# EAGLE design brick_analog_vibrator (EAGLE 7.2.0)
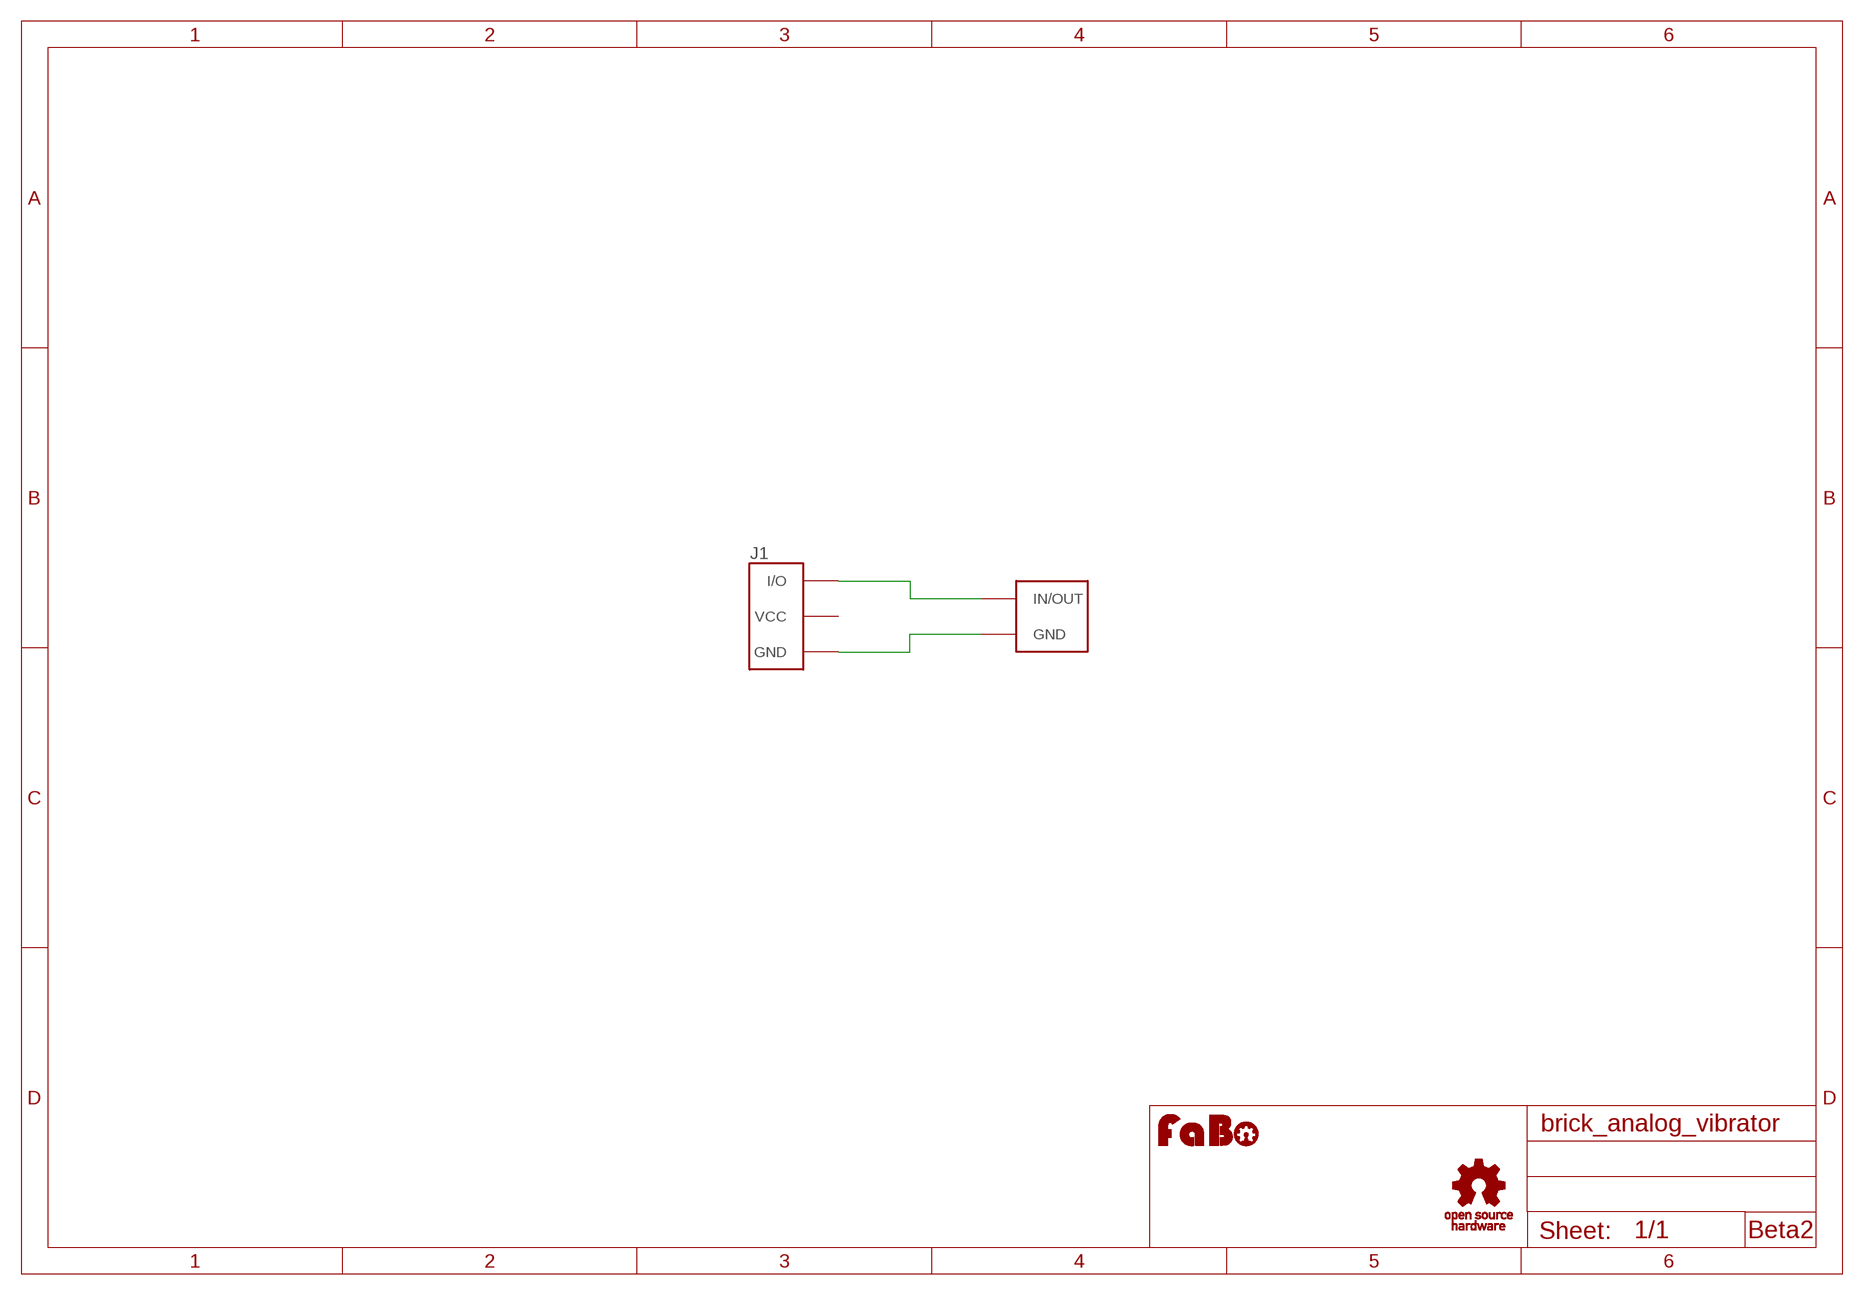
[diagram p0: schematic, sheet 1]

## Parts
J1  BRICK_3PIN  [BRICK_3PIN]
U1  LA3R5-480H1-PTH  [LA3R5-480AH1_PTH]
U$1  LOGO_FABO-M  [LOGO_FABO_M]
U$5  LOGO_OSHW_T-M  [LOGO_OSHW_T_M]

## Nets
GND: J1.GND U1.P$2(GND)
N$1: J1.IN/OUT(I/O) U1.P$1(IN/OUT)
Unconnected: J1.VCC

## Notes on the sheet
- Beta2

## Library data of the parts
J1 = gclue:BRICK_3PIN: FaBo Brick 3pin
U1 = gclue:LA3R5-480H1
U$1 = FaBo:LOGO_FABO
U$5 = gclue:LOGO_OSHW_T

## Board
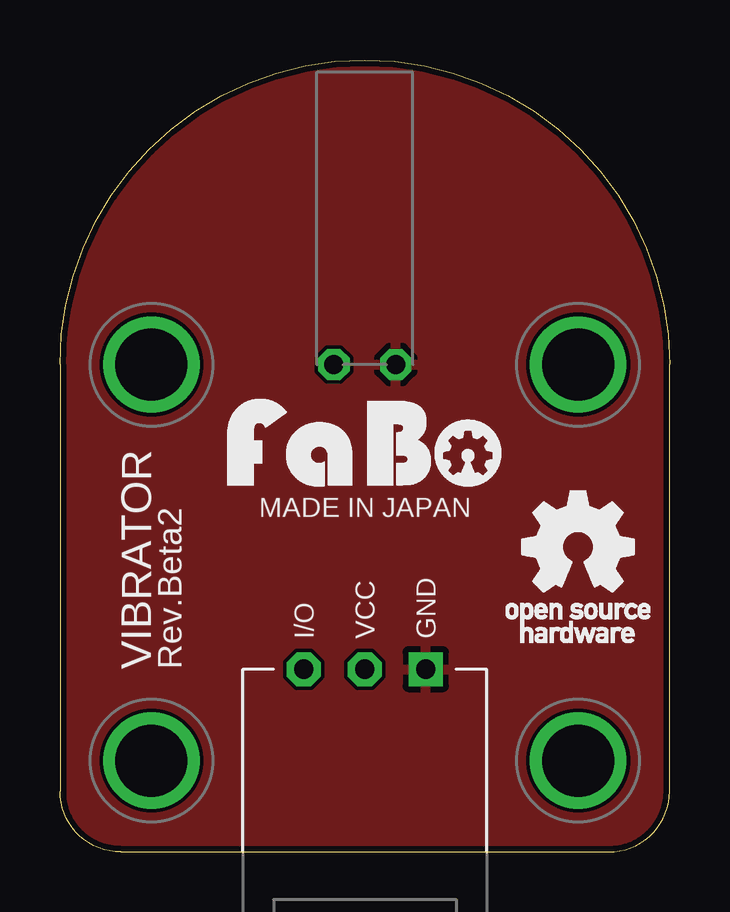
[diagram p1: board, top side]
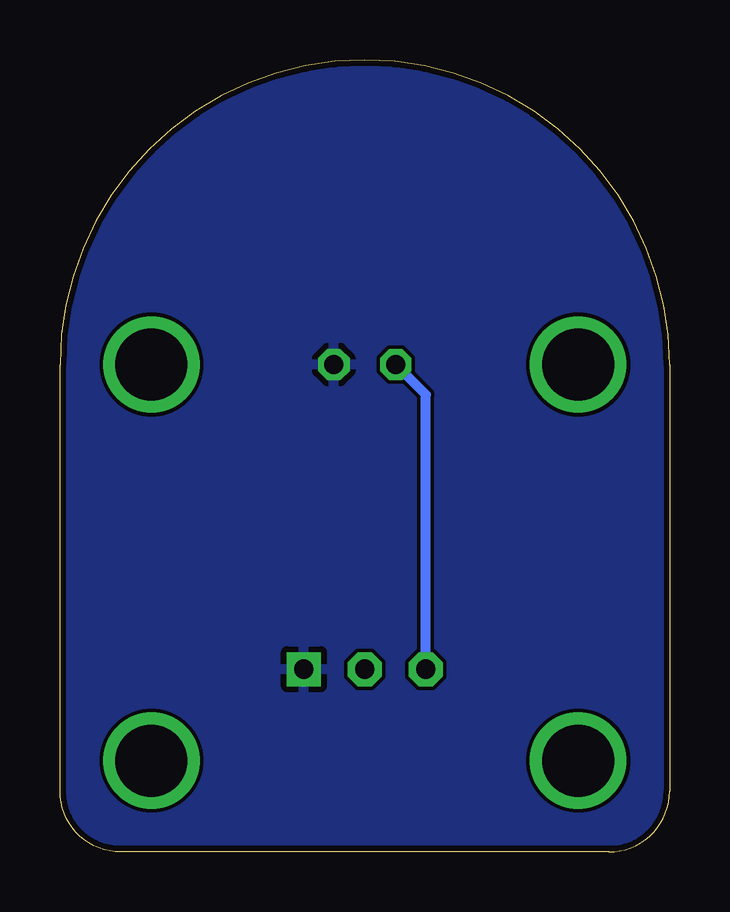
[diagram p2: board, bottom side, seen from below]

Size 25.4 x 33.02 mm. Coordinates in mm from the lower left corner, seen from the top.
Copper layers (1*16): Top 0.035mm / dielectric 1.5mm / Bottom 0.035mm
Design rules "Elecrow_2-layer_eagle_rule": minimum track width 6mil, minimum drill 12mil, track to track 6mil, track to pad 6mil, pad to pad 6mil, via to via 6mil, smd to smd 0mil, copper to edge 10mil, drill to drill 10mil, minimum pad ring 10mil, minimum via ring 6mil, stop-mask expansion 2mil, vias tented up to drill 100mil, thermal gap 10mil

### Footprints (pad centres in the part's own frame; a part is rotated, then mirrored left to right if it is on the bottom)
BRICK_3PIN = drill 0.8 pad 1.422 square: GND 2.54,-8.89 | drill 0.8 pad 1.422 octagon: IN/OUT -2.54,-8.89; VCC 0,-8.89 | drill 3 pad 3.81: P$5 -8.89,3.81; P$6 8.89,3.81; P$7 -8.89,-12.7; P$8 8.89,-12.7
LA3R5-480AH1_PTH = drill 0.8 octagon: P$1 -1.29,0; P$2 1.29,0

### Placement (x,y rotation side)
J1  12.7,16.51 0 top
U1  12.7,20.32 0 top
U$1  12.7,15.24 0 top
U$5  21.59,12.7 0 top

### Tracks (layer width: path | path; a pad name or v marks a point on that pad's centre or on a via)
GND
  pour Bottom: -1.27,-1.27 26.67,-1.27 26.67,34.29 -1.27,34.29
  pour Top: -1.27,-1.27 26.67,-1.27 26.67,34.29 -1.27,34.29
N$1
  Bottom 0.406: J1.IN/OUT 10.16,19.07 U1.P$1

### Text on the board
tPlace: MADE IN JAPAN | VIBRATOR | Rev.Beta2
